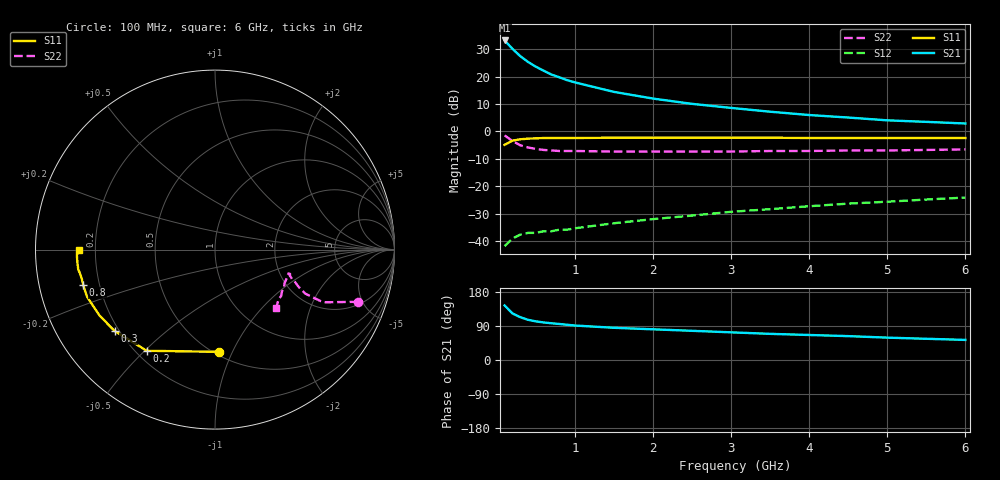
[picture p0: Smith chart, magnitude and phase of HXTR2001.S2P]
! HXTR-2001 Common Emitter
! Vce=15V  Ic=25mA
# ghz s ma r 50
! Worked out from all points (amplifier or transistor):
!   20 points, 100 MHz to 6 GHz, reference 50 ohm
!   highest |S21| = 33.3 dB at 100 MHz (marker M1)
!   |S21| within 3 dB of that: start of sweep to 198.2 MHz
!   unconditionally stable (mu >= 1): 865.7 MHz to end of sweep
!   at 400 MHz: K = 0.50, MSG = 31.3 dB, |S12| = -37.1 dB
!   at 1.5 GHz: K = 1.28, MAG = 20.9 dB, |S12| = -33.6 dB
!   at 6 GHz: K = 1.61, MAG = 9.0 dB, |S12| = -24.2 dB
!   S11 on the Smith chart (normalised r, x): 100 MHz: 0.53, -0.89; 200 MHz: 0.24, -0.51; 300 MHz: 0.18, -0.34; 800 MHz: 0.14, -0.13; 6 GHz: 0.14, -0.00
0.1  0.57 -88.0  46.2 144.0  0.008 58.0  0.85 -20.0
0.2  0.68 -124.0  32.5 123.0  0.011 43.0  0.67 -26.0
0.3  0.72 -141.0  23.9 113.0  0.013 37.0  0.56 -26.0
0.4  0.74 -150.0  18.7 106.0  0.014 35.0  0.51 -24.0
0.5  0.75 -156.0  15.3 102.0  0.014 35.0  0.48 -22.0
0.6  0.76 -160.0  12.9 99.0  0.015 36.0  0.46 -21.0
0.7  0.76 -163.0  11 97.0  0.015 37.0  0.45 -20.0
0.8  0.76 -165.0  9.8 95.0  0.016 38.0  0.44 -19.0
0.9  0.76 -167.0  8.7 93.0  0.016 40.0  0.44 -18.0
1  0.76 -168.0  7.9 91.0  0.017 42.0  0.44 -18.0
1.5  0.77 -172.0  5.3 85.0  0.021 49.0  0.43 -18.0
2  0.77 -175.0  4 81.0  0.025 54.0  0.43 -20.0
2.5  0.77 -176.0  3.2 77.0  0.029 58.0  0.43 -23.0
3  0.77 -177.0  2.7 73.0  0.034 60.0  0.43 -26.0
3.5  0.77 -178.0  2.3 69.0  0.038 61.0  0.44 -29.0
4  0.76 -179.0  2 66.0  0.043 62.0  0.44 -32.0
4.5  0.76 -179.0  1.8 63.0  0.048 62.0  0.45 -35.0
5  0.76 -179.0  1.6 59.0  0.052 62.0  0.45 -38.0
5.5  0.76 -180.0  1.5 56.0  0.057 62.0  0.46 -41.0
6  0.76 -180.0  1.4 53.0  0.062 61.0  0.47 -44.0
